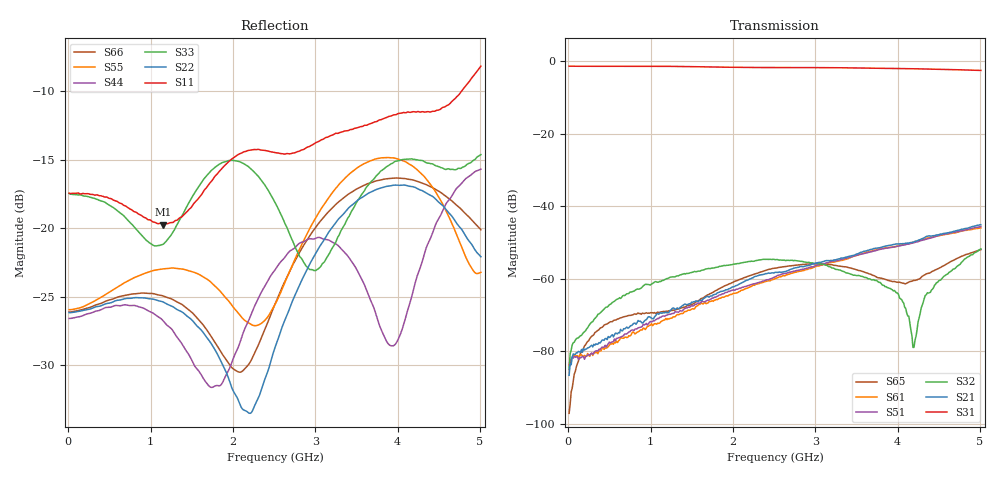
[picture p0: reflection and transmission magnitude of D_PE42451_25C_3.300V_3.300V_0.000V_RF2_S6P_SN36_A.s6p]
! Device ID: PE42451
! Serial: 36
! Insertion: A
! Temp: 25C
! VDD: 3.300
! Control_Hi: 100.000
! Control_Lo: 0.000
! Logic State: RF2
! Port 1: RFC
! Port 2: RF1
! Port 3: RF2
! Port 4: RF3
! Port 5: RF4
! Port 6: RF5
! V1 = 0.00
! V2 = 3.30
! V3 = 0.00
! V4 = 0.00
! IDD: 1.621010e-05
#  Hz  S  RI  R  50
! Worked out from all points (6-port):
!   401 points, 10 MHz to 5.01 GHz, reference 50 ohm
!   strongest paths, dB at 10 MHz, 1.26 GHz, 2.51 GHz, 3.76 GHz, 5.01 GHz:
!     S31: -1.4, -1.4, -1.8, -1.9, -2.5
!     S21: -86.6, -68.2, -58.2, -51.5, -45.1
!     S32: -84.8, -59.5, -54.7, -60.8, -51.8
!     S51: -85.0, -69.6, -59.4, -52.0, -45.6
!     S61: -83.8, -70.8, -60.0, -51.8, -46.0
!     S65: -97.1, -68.7, -57.0, -59.7, -51.9
!   lowest |S11| = -19.7 dB at 1.147 GHz (marker M1), VSWR 1.23, Z = 57.3 - j8.4 ohm
!   |S11| at or under -10 dB: start of sweep to 4.772 GHz
